PROGRAM main
VAR
	push_ratio AT %Q*: USINT :=50;					//Object 201Ah 1h: Push Mode(SUbIndex:1h Push ratio)
	pull_back AT %Q*: UDINT :=100;					//Object 201Ah 2h: Push Mode(SUbIndex:2h Pull back destance)
	control_word AT %Q*: UINT :=0;					//Object 6040h: Control Word
	status_word AT %I*: UINT;						//Object 6041h: Status Word
	mode_of_operation AT %Q*: SINT :=0;				//Object 6061h: Mode of Operation 1:pp mode 6:home mode 8:csp mode
	target_position AT %Q*: DINT :=100000;			//Object 607Ah: Target position
	profile_velocity AT %Q*: UDINT :=10000;			//Object 6081h: Profile Velocity
	profile_acceleration AT %Q*: UDINT :=100000;	//Object 6083h: Profile Acceleration
	profile_deceleration AT %Q*: UDINT :=100000;	//Object 6084h: Profile Deceleration
	
	error_code AT %I*: UINT;						//Object 603fh: Erroe Code
	actual_pos AT %I*: DINT;						//Object 6064h: Position Actual Value
	actual_vel AT %I*: DINT;						//Object 606bh: Velocity Demand Value
	position_demand_value AT %I*: DINT;				//Object 6062h: Position Demand Value
	following_erroe_actual_value AT %I*: DINT;		//Object 60F4h: Following Erroe Actual Value

	homing_method AT %Q*: SINT :=0;					//Object 6098h: Homing method
//	homing_speed AT %Q*: UDINT :=5000;				//Object 6099h 1h: Homing Speeds(SUbIndex:2h Speed)
//	homing_acceleration AT %Q*: UDINT :=100000;		//Object 609Ah: Homing Acceleration
//	homing_torque_raito AT %Q*: USINT;				//Object 6014h: Homing Torque Raito
//	homing_offset AT %Q*: DINT;						//Object 607Ch: Homing Offset
//	polarity AT %Q*: USINT;							//Object 607Eh: Polarity
	
	cmd_pos_count: DINT;
	act_pos_count: DINT;
	pos_error_count: DINT;
	
	pos_reset: BOOL;
	cmd_pos_counta: DINT :=0;
	act_pos_counta: DINT :=0;
	pos_error_counta: DINT :=0;
	
	digital_input AT %I*: UDINT;					//Object 60FDh: Digital Input
	digital_output AT %Q*: UDINT :=0;				//Object 60FEh 1h: DIgital Output
	limit_m: UDINT;
	limit_p: UDINT;
	org0: UDINT;
	lim_m: BOOL;
	lim_p: BOOL;
	org: BOOL;
	z_pulse: BOOL;
	z0: UDINT;
	
	in1: BOOL;
	in2: BOOL;
	in3: BOOL;
	in4: BOOL;
	in5: BOOL;
	in6: BOOL;
	in1a: UDINT;
	in2a: UDINT;
	in3a: UDINT;
	in4a: UDINT;
	in5a: UDINT;
	in6a: UDINT;
	
	out1: BOOL;
	out2: BOOL;
	out3: BOOL;
	out4: BOOL;
	out5: BOOL;	
	out1a: UDINT;
	out2a: UDINT;
	out3a: UDINT;
	out4a: UDINT;
	out5a: UDINT;
	
	enable_on: BOOL;
	enable_off: BOOL;
	enable: UINT :=16#0006;
	enable_set: UINT;
	enable_ope: BOOL;
	enable_ope_n: BOOL;
	
	move_frame_sel: BYTE :=0;	
	
	stop_dec: BOOL;
	SDO_Write01: FB_EcCoESdoWrite;
	stop_set: UINT;
	stop_imm: BOOL;
	stop_imm_r: BOOL;
	stop_dec_r: BOOL;
	stop_r_set: BOOL;
	
	mode_of_ope: BYTE :=0;
	axis_move: BOOL;
	axis_stop: BOOL;
	target_reached: UINT;	
	alarm_reset_sw: BOOL;
	alarm_reset: UINT;
	sw_p_limit: BOOL;
	sw_n_limit: BOOL;
	inposition: BOOL;
	drive_error: BOOL;
	push_state: UINT;
	push_detected: UINT;
	push_detected_led: BOOL;
	push_state_led: BOOL;
	org_returning: UINT;
	org_ret: UINT;
	org_returning_led: BOOL;
	org_ret_led: BOOL;
	motioning: UINT;
	motioning_led: BOOL;
	motion_dir_led: BOOL;
	Safty_act: UINT;
	Safty_act_led: BOOL;
	velocity: UDINT;
	motion_const_led: BOOL;
	motion_accel_led: BOOL;;
	motion_decel_led: BOOL;
	actual_vel_back: UDINT;
	FB_EcCoESdoRead_0: FB_EcCoESdoRead;
	read_data: DINT;;
	actual_vela: DINT;
	actual_velb: UDINT;
	TON_0: TON;
END_VAR
VAR // added by the converter: edge detectors and wires of the graphical bodies
    _w1, _w2, _w3, _w4, _w5, _w6, _w7, _w8, _w9 : BOOL;
END_VAR

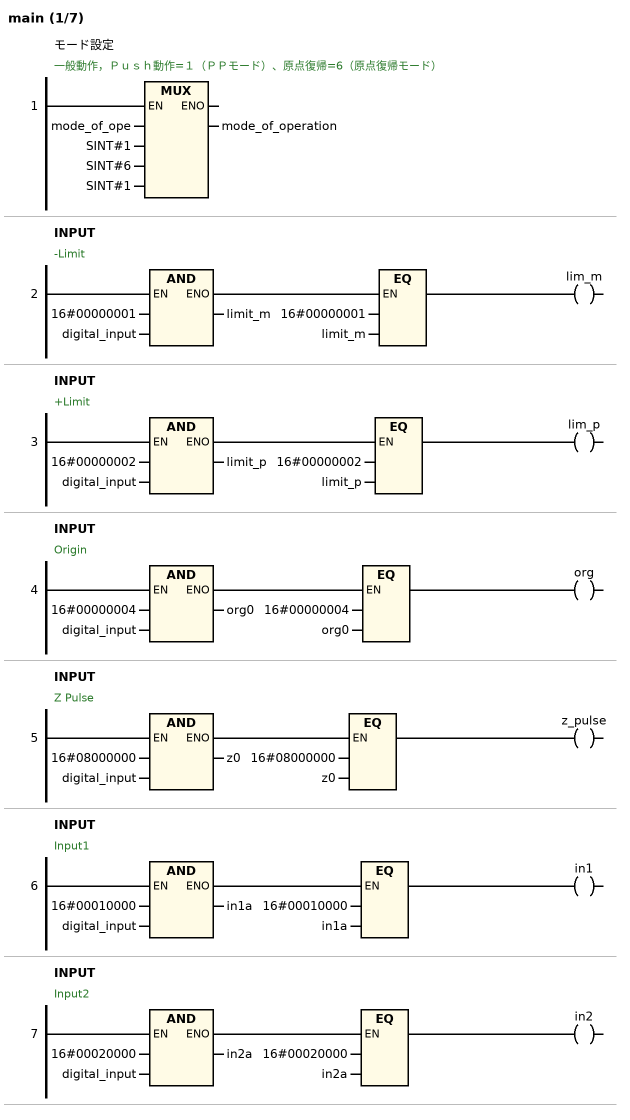
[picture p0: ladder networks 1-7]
// NETWORK 1: モード設定
// 一般動作，Ｐｕｓｈ動作=１（ＰＰモード）、原点復帰=6（原点復帰モード）
mode_of_operation := MUX(mode_of_ope, SINT#1, SINT#6, SINT#1);

// NETWORK 2: INPUT
// -Limit
limit_m := 16#00000001 AND digital_input;
lim_m := 16#00000001 = limit_m;

// NETWORK 3: INPUT
// +Limit
limit_p := 16#00000002 AND digital_input;
lim_p := 16#00000002 = limit_p;

// NETWORK 4: INPUT
// Origin
org0 := 16#00000004 AND digital_input;
org := 16#00000004 = org0;

// NETWORK 5: INPUT
// Z Pulse
z0 := 16#08000000 AND digital_input;
z_pulse := 16#08000000 = z0;

// NETWORK 6: INPUT
// Input1
in1a := 16#00010000 AND digital_input;
in1 := 16#00010000 = in1a;

// NETWORK 7: INPUT
// Input2
in2a := 16#00020000 AND digital_input;
in2 := 16#00020000 = in2a;

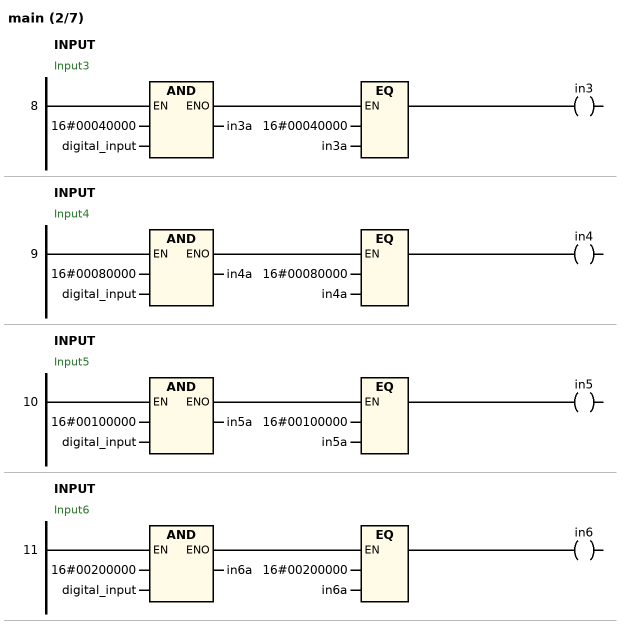
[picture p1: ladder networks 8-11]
// NETWORK 8: INPUT
// Input3
in3a := 16#00040000 AND digital_input;
in3 := 16#00040000 = in3a;

// NETWORK 9: INPUT
// Input4
in4a := 16#00080000 AND digital_input;
in4 := 16#00080000 = in4a;

// NETWORK 10: INPUT
// Input5
in5a := 16#00100000 AND digital_input;
in5 := 16#00100000 = in5a;

// NETWORK 11: INPUT
// Input6
in6a := 16#00200000 AND digital_input;
in6 := 16#00200000 = in6a;

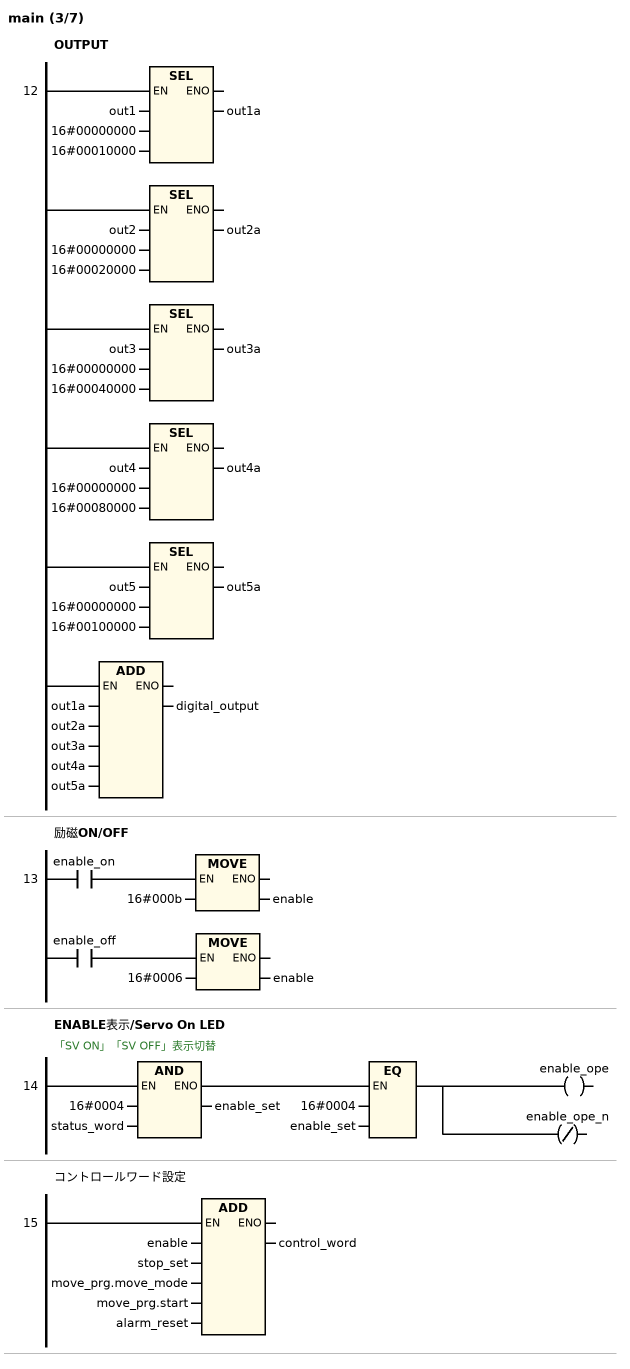
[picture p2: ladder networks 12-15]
// NETWORK 12: OUTPUT
out1a := SEL(out1, 16#00000000, 16#00010000);
out2a := SEL(out2, 16#00000000, 16#00020000);
out3a := SEL(out3, 16#00000000, 16#00040000);
out4a := SEL(out4, 16#00000000, 16#00080000);
out5a := SEL(out5, 16#00000000, 16#00100000);
digital_output := out1a + out2a + out3a + out4a + out5a;

// NETWORK 13: 励磁ON/OFF
IF enable_on THEN enable := 16#000b; END_IF
IF enable_off THEN enable := 16#0006; END_IF

// NETWORK 14: ENABLE表示/Servo On LED
// 「SV ON」「SV OFF」表示切替
enable_set := 16#0004 AND status_word;
_w1 := 16#0004 = enable_set;
enable_ope := _w1;
enable_ope_n := NOT _w1;

// NETWORK 15: コントロールワード設定
control_word := enable + stop_set + move_prg.move_mode + move_prg.start + alarm_reset;

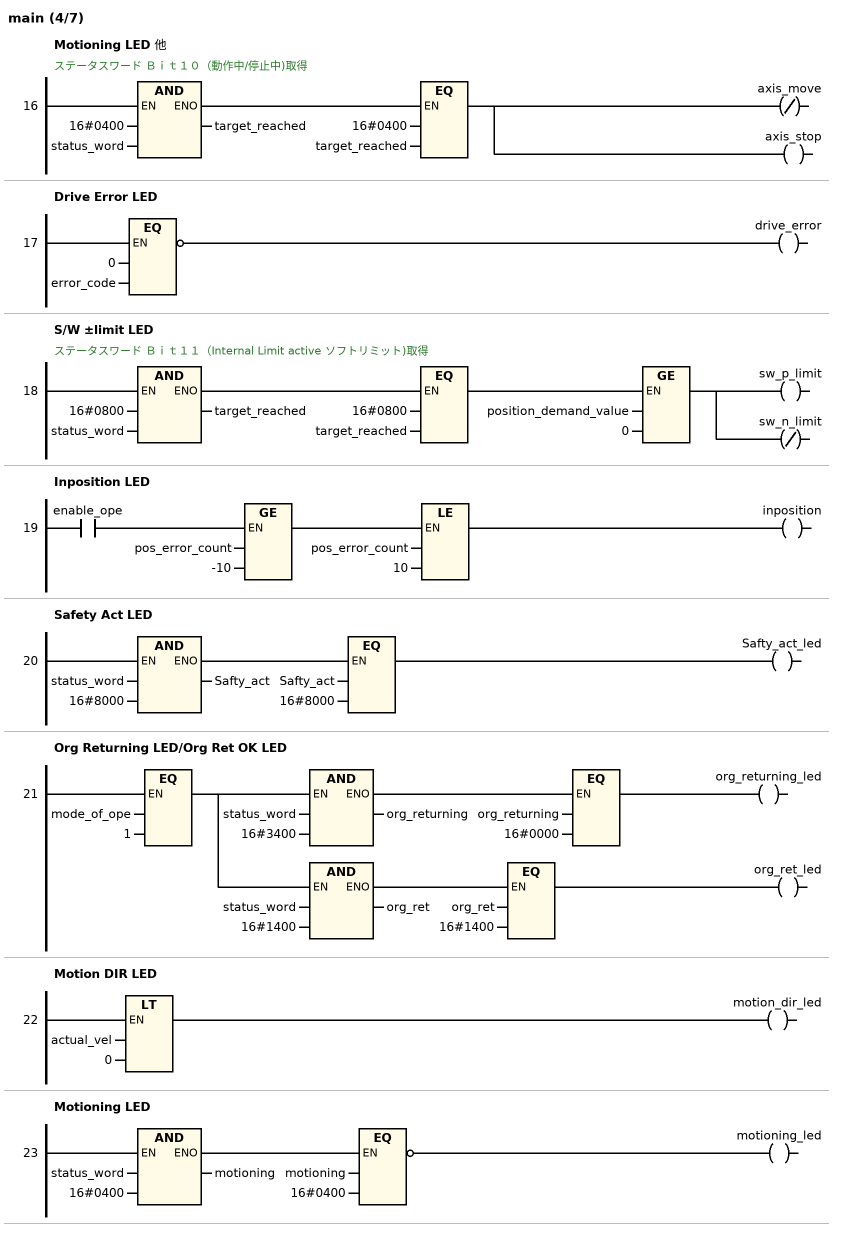
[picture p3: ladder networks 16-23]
// NETWORK 16: Motioning LED 他
// ステータスワード Ｂｉｔ１０（動作中/停止中)取得
target_reached := 16#0400 AND status_word;
_w2 := 16#0400 = target_reached;
axis_move := NOT _w2;
axis_stop := _w2;

// NETWORK 17: Drive Error LED
drive_error := NOT (0 = error_code);

// NETWORK 18: S/W ±limit LED
// ステータスワード Ｂｉｔ１１（Internal Limit active ソフトリミット)取得
target_reached := 16#0800 AND status_word;
_w3 := 16#0800 = target_reached AND position_demand_value >= 0;
sw_p_limit := _w3;
sw_n_limit := NOT _w3;

// NETWORK 19: Inposition LED
inposition := enable_ope AND pos_error_count >= -10 AND pos_error_count <= 10;

// NETWORK 20: Safety Act LED
Safty_act := status_word AND 16#8000;
Safty_act_led := Safty_act = 16#8000;

// NETWORK 21: Org Returning LED/Org Ret OK LED
_w4 := mode_of_ope = 1;
IF _w4 THEN org_returning := status_word AND 16#3400; END_IF
org_returning_led := _w4 AND org_returning = 16#0000;
IF _w4 THEN org_ret := status_word AND 16#1400; END_IF
org_ret_led := _w4 AND org_ret = 16#1400;

// NETWORK 22: Motion DIR LED
motion_dir_led := actual_vel < 0;

// NETWORK 23: Motioning LED
motioning := status_word AND 16#0400;
motioning_led := NOT (motioning = 16#0400);

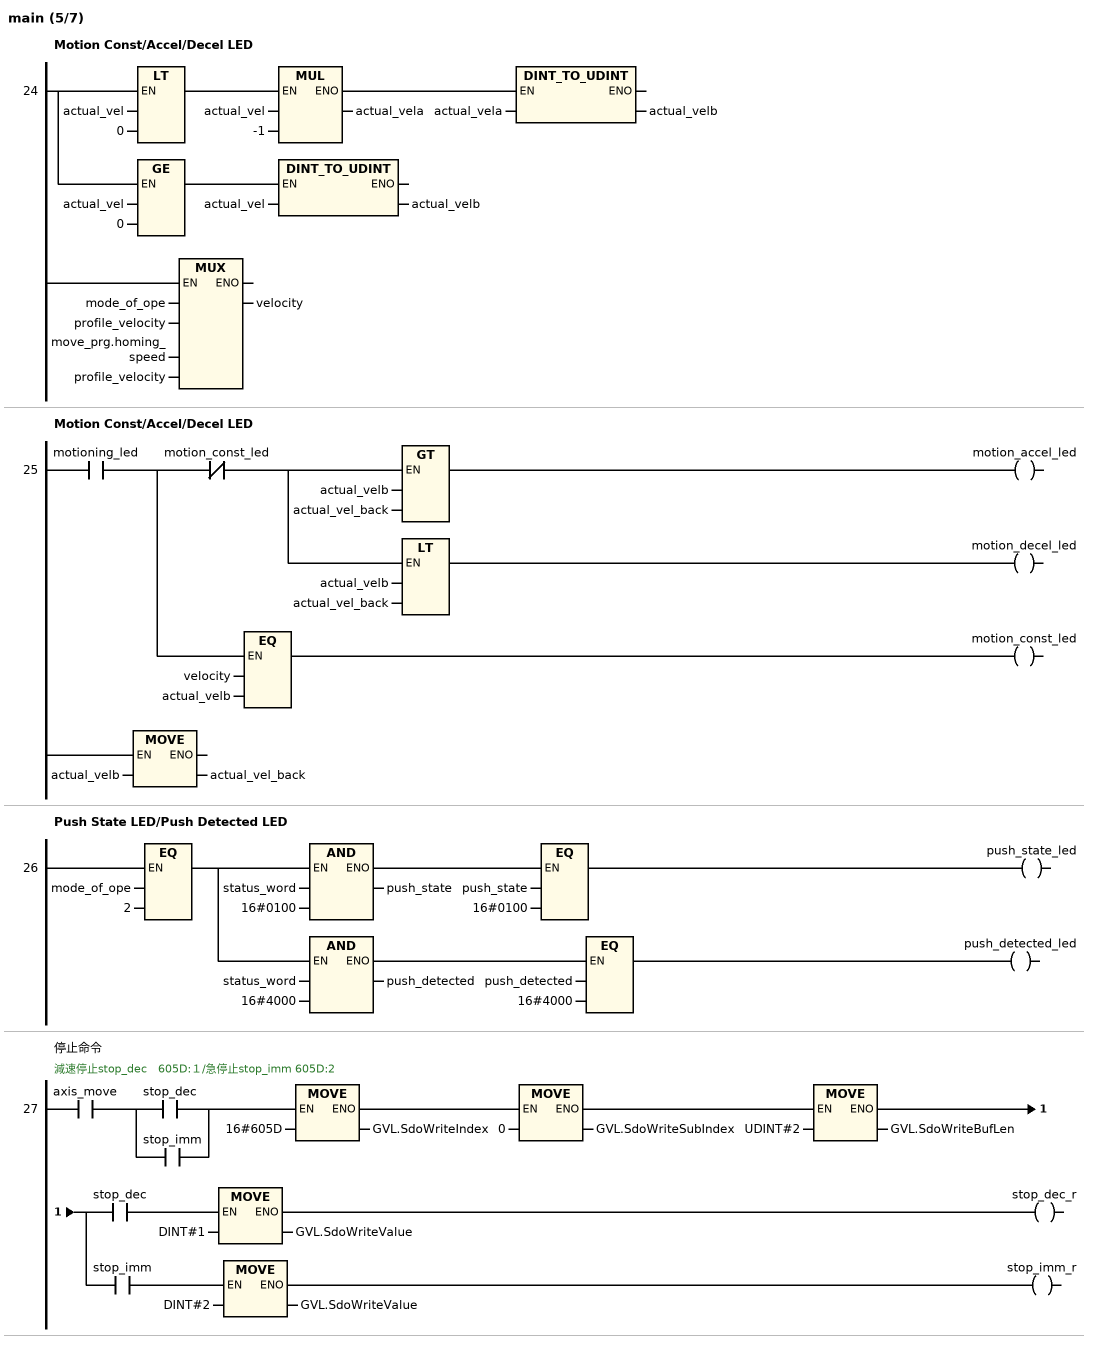
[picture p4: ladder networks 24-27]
// NETWORK 24: Motion Const/Accel/Decel LED
_w5 := actual_vel < 0;
IF _w5 THEN actual_vela := actual_vel * -1; END_IF
IF _w5 THEN actual_velb := DINT_TO_UDINT(actual_vela); END_IF
IF actual_vel >= 0 THEN actual_velb := DINT_TO_UDINT(actual_vel); END_IF
velocity := MUX(mode_of_ope, profile_velocity, move_prg.homing_speed, profile_velocity);

// NETWORK 25: Motion Const/Accel/Decel LED
_w6 := motioning_led AND NOT motion_const_led;
motion_accel_led := _w6 AND actual_velb > actual_vel_back;
motion_decel_led := _w6 AND actual_velb < actual_vel_back;
motion_const_led := motioning_led AND velocity = actual_velb;
actual_vel_back := actual_velb;

// NETWORK 26: Push State LED/Push Detected LED
_w7 := mode_of_ope = 2;
IF _w7 THEN push_state := status_word AND 16#0100; END_IF
push_state_led := _w7 AND push_state = 16#0100;
IF _w7 THEN push_detected := status_word AND 16#4000; END_IF
push_detected_led := _w7 AND push_detected = 16#4000;

// NETWORK 27: 停止命令
// 減速停止stop_dec　605D:１/急停止stop_imm 605D:2
_w8 := axis_move AND (stop_dec OR stop_imm);
IF _w8 THEN GVL.SdoWriteIndex := 16#605D; END_IF
IF _w8 THEN GVL.SdoWriteSubIndex := 0; END_IF
IF _w8 THEN GVL.SdoWriteBufLen := UDINT#2; END_IF
IF _w8 AND stop_dec THEN GVL.SdoWriteValue := DINT#1; END_IF
stop_dec_r := _w8 AND stop_dec;
IF _w8 AND stop_imm THEN GVL.SdoWriteValue := DINT#2; END_IF
stop_imm_r := _w8 AND stop_imm;

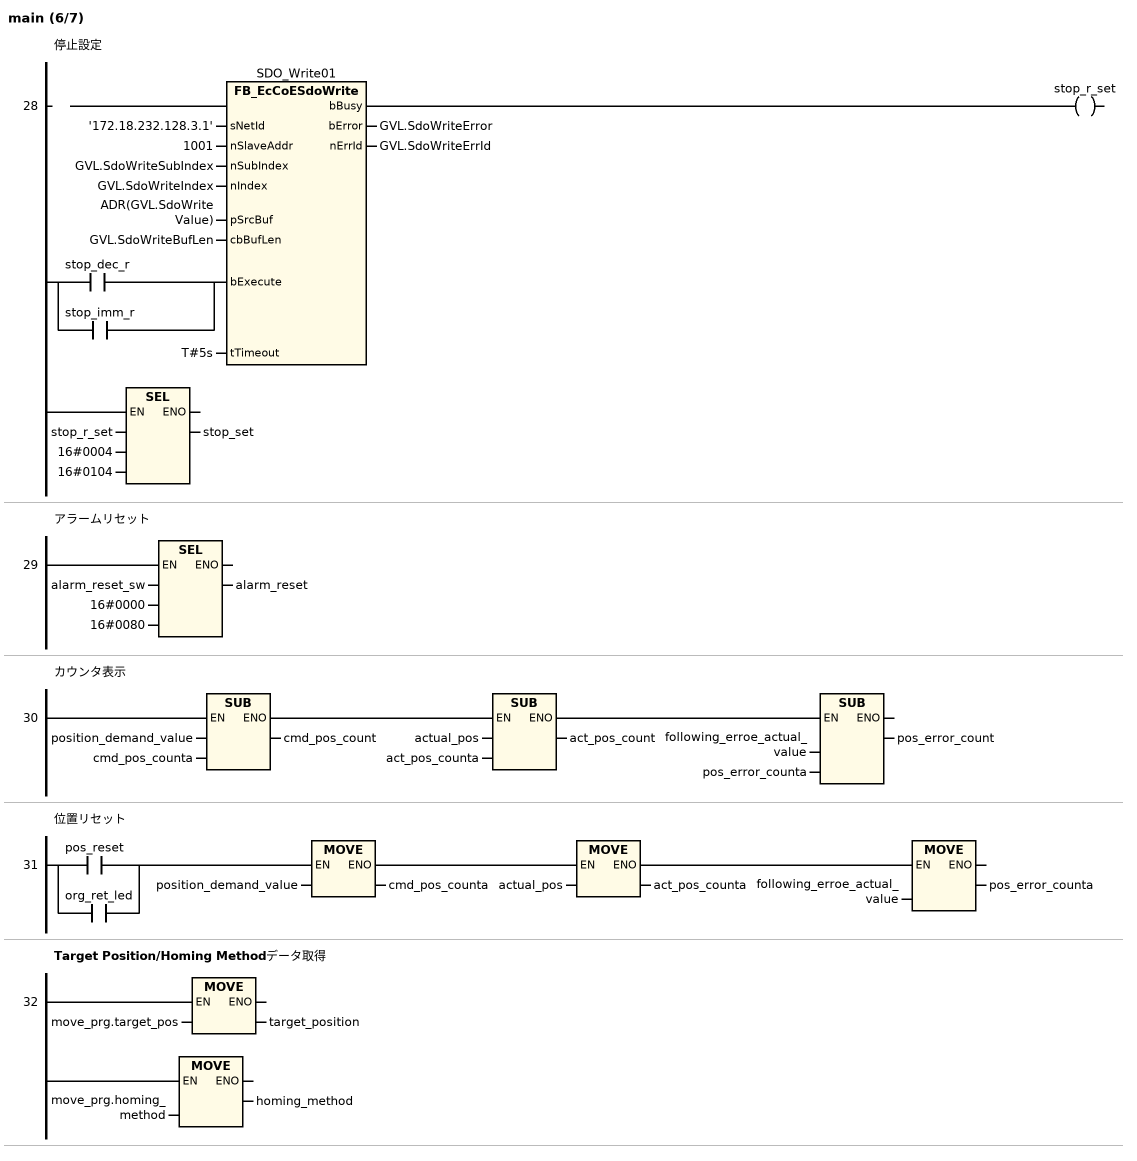
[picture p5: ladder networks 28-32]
// NETWORK 28: 停止設定
SDO_Write01(
    sNetId := '172.18.232.128.3.1',
    nSlaveAddr := 1001,
    nSubIndex := GVL.SdoWriteSubIndex,
    nIndex := GVL.SdoWriteIndex,
    pSrcBuf := ADR(GVL.SdoWriteValue),
    cbBufLen := GVL.SdoWriteBufLen,
    bExecute := stop_dec_r OR stop_imm_r,
    tTimeout := T#5s,
    bError => GVL.SdoWriteError,
    nErrId => GVL.SdoWriteErrId); // FB_EcCoESdoWrite
stop_r_set := SDO_Write01.bBusy;
stop_set := SEL(stop_r_set, 16#0004, 16#0104);

// NETWORK 29: アラームリセット
alarm_reset := SEL(alarm_reset_sw, 16#0000, 16#0080);

// NETWORK 30: カウンタ表示
cmd_pos_count := position_demand_value - cmd_pos_counta;
act_pos_count := actual_pos - act_pos_counta;
pos_error_count := following_erroe_actual_value - pos_error_counta;

// NETWORK 31: 位置リセット
_w9 := pos_reset OR org_ret_led;
IF _w9 THEN cmd_pos_counta := position_demand_value; END_IF
IF _w9 THEN act_pos_counta := actual_pos; END_IF
IF _w9 THEN pos_error_counta := following_erroe_actual_value; END_IF

// NETWORK 32: Target Position/Homing Methodデータ取得
target_position := move_prg.target_pos;
homing_method := move_prg.homing_method;

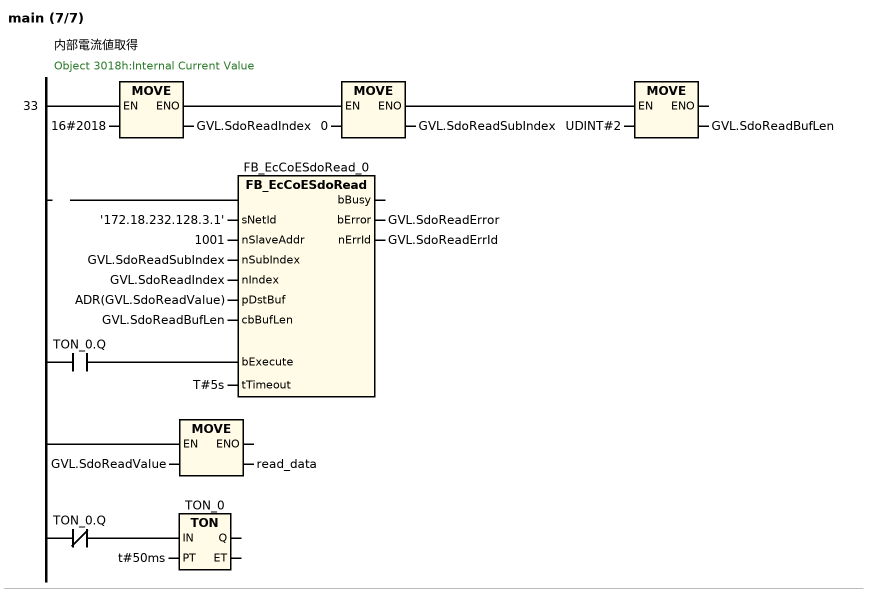
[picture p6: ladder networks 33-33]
// NETWORK 33: 内部電流値取得
// Object 3018h:Internal Current Value
GVL.SdoReadIndex := 16#2018;
GVL.SdoReadSubIndex := 0;
GVL.SdoReadBufLen := UDINT#2;
FB_EcCoESdoRead_0(
    sNetId := '172.18.232.128.3.1',
    nSlaveAddr := 1001,
    nSubIndex := GVL.SdoReadSubIndex,
    nIndex := GVL.SdoReadIndex,
    pDstBuf := ADR(GVL.SdoReadValue),
    cbBufLen := GVL.SdoReadBufLen,
    bExecute := TON_0.Q,
    tTimeout := T#5s,
    bError => GVL.SdoReadError,
    nErrId => GVL.SdoReadErrId); // FB_EcCoESdoRead
read_data := GVL.SdoReadValue;
TON_0(IN := NOT TON_0.Q, PT := t#50ms); // TON

END_PROGRAM
